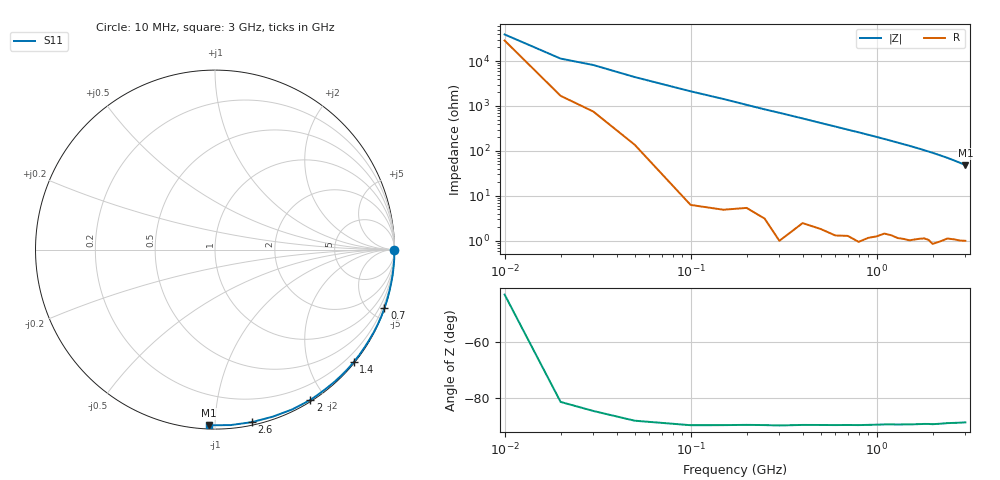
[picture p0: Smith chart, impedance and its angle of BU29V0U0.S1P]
! SIEMENS Small Signal Semiconductors
! BB833
! Si Tuning Diode in SOD323
! VR = 29 V
! S-Parameters:  April  1996
# GHz  S  MA  R  50
!  f  S11
! GHz  MAG  ANG
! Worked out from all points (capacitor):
!   31 points, 10 MHz to 3 GHz, reference 50 ohm
!   read as one part to ground: C = 654 fF near 10 MHz
!   lowest |Z| = 48.2 ohm at 3 GHz (marker M1)
!   S11 on the Smith chart (normalised r, x): 10 MHz: open; 700 MHz: 0.03, -5.94; 1.4 GHz: 0.02, -2.82; 2 GHz: 0.02, -1.82; 2.6 GHz: 0.02, -1.24; 3 GHz: 0.02, -0.96
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0.01  0.9981 -0.1
0.02  0.9987 -0.5
0.03  0.9989 -0.7
0.1  0.9999 -2.7
0.15  0.9998 -4.0
0.25  0.9996 -6.8
0.3  0.9998 -8.1
0.4  0.9991 -10.8
0.5  0.999 -13.6
0.6  0.9989 -16.3
0.7  0.9986 -19.1
0.8  0.9986 -21.8
0.9  0.9979 -24.6
1  0.9972 -27.4
1.2  0.9957 -33.2
1.3  0.9956 -36.2
1.4  0.9951 -39.1
1.5  0.9947 -42.0
1.6  0.9937 -45.1
1.7  0.9926 -48.1
1.8  0.9915 -51.3
1.9  0.9912 -54.5
2  0.9921 -57.6
2.2  0.989 -64.2
2.4  0.9849 -70.9
2.6  0.983 -77.9
2.8  0.9816 -84.9
3  0.9794 -92.1
